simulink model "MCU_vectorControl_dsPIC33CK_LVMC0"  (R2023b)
settings: Solver=FixedStepDiscrete  StartTime=0.0  StopTime=10.0  FixedStep=5e-5  RelTol=1e-3  EnableMultiTasking=on
undefined symbols (not defined in the file or in its folder): A0, A4, ADC, address, also, AN0, AN1, as, B0, B2, below, Bias1, Bias2, bit, bits, BOR, C12, C13, C14, C7, C8, cause, Code, Communicate, control, counter, Custom, D11, D12, D13, D14, D2, D5, D6, D7, D9, dead, default, deviced, diff, disasserted, DiscIntNeverNeededParam, ECIO, ensure, events, faster, HS3, I, I2C, I2C1, I2C2, I2C3, illegalInstruction, Interval, inverter, is, IsSigned1, IsSigned2, kHz, Lowest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
libraries: simulink x55, MCHP_Blockset x25
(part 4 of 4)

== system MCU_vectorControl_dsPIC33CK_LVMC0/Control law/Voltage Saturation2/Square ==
  In1 : Inport
  Data Type Propagation : simulink/Signal Attributes/Data Type Propagation  PropDataType=fixdt(1, 16)  IfRefDouble=double  IfRefSingle=single  IsSigned=IsSigned1 or IsSigned2  NumBitsBase=max([NumBits1 NumBits2])  NumBitsMult=1  NumBitsAdd=0  NumBitsAllowFinal=1:128  PropScalingMode=Specify via dialog  PropScaling=2^-model.FracLen.volt2  ValuesUsedBestPrec=[5 -7]  SlopeBase=PosRange1*PosRange2  SlopeMult=1  SlopeAdd=0  BiasBase=max([Bias1 Bias2])  BiasMult=1  BiasAdd=0
  Square : Math  Operator=square  OutDataTypeStr=Inherit: Inherit via back propagation
  y : Outport
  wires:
  Square/1 -> Data Type Propagation/3, y/1
  In1/1 -> Square/1, Data Type Propagation/2, Data Type Propagation/1

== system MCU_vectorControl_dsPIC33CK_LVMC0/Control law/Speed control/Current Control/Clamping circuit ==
  note: The clamping enable or disable the integral action.
  preIntegrator : Inport  DisableCoverage=on
  saturation : Inport  DisableCoverage=on  Port=2
  AND : Logic  Operator=OR  IconShape=distinctive  AllPortsSameDT=off  OutDataTypeStr=boolean
  Compare To Zero1 : simulink/Logic and Bit Operations/Compare To Zero  relop=<=  OutDataTypeStr=boolean
  Delay : Delay  DelayLength=1
  Demux : Demux  Outputs=2
  Multiply : Product
  Clamp : Outport  DisableCoverage=on  VectorParamsAs1DForOutWhenUnconnected=off
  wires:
  saturation/1 -> Delay/1
  Compare To Zero1/1 -> Demux/1
  Multiply/1 -> Compare To Zero1/1
  preIntegrator/1 -> Multiply/2
  AND/1 -> Clamp/1
  Demux/2 -> AND/2
  Demux/1 -> AND/1
  Delay/1 -> Multiply/1

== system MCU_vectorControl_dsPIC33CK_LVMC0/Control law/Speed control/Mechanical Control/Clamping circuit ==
  note: The clamping enable or disable the integral action.
  Saturation : Inport  DisableCoverage=on
  preIntegrator : Inport  DisableCoverage=on  Port=2
  Compare To Zero1 : simulink/Logic and Bit Operations/Compare To Zero  relop=<=  OutDataTypeStr=boolean
  Delay : Delay  DelayLength=1  InitialCondition=0
  Multiply : Product
  Clamp : Outport  DisableCoverage=on  VectorParamsAs1DForOutWhenUnconnected=off
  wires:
  Delay/1 -> Multiply/1
  Saturation/1 -> Delay/1
  Multiply/1 -> Compare To Zero1/1
  preIntegrator/1 -> Multiply/2
  Compare To Zero1/1 -> Clamp/1

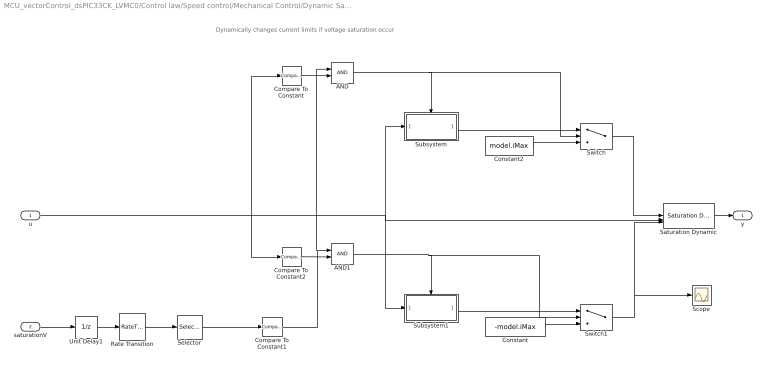
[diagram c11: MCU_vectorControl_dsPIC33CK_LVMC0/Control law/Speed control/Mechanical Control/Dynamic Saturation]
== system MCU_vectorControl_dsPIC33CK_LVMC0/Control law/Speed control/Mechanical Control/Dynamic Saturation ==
  note: Dynamically changes current limits if voltage saturation occur
  u : Inport
  saturationV : Inport  Port=2
  AND : Logic  IconShape=distinctive  AllPortsSameDT=off  OutDataTypeStr=boolean
  AND1 : Logic  IconShape=distinctive  AllPortsSameDT=off  OutDataTypeStr=boolean
  Compare To Constant : simulink/Logic and Bit Operations/Compare To Constant  relop=>=  const=0  OutDataTypeStr=boolean
  Compare To Constant1 : simulink/Logic and Bit Operations/Compare To Constant  relop=~=  const=0  OutDataTypeStr=boolean
  Compare To Constant2 : simulink/Logic and Bit Operations/Compare To Constant  relop=<  const=0  OutDataTypeStr=boolean
  Constant : Constant  Value=-model.iMax  OutDataTypeStr=single  SampleTime=1e-3
  Constant2 : Constant  Value=model.iMax  OutDataTypeStr=single  SampleTime=1e-3
  Rate Transition : RateTransition  OutPortSampleTime=control.tsMeca
  Saturation Dynamic : simulink/Discontinuities/Saturation Dynamic  OutMin=[]  OutMax=[]  OutDataTypeStr=Inherit: Same as second input  OutDataType=fixdt(1, 16)  OutScaling=2^-10  DoSatur=off
  Scope : Scope
  Selector : Selector  InputPortWidth=2  IndexOptions=Index vector (dialog)  Indices=2  OutputSizes=1
  Subsystem : Subsystem
  Subsystem1 : Subsystem
  Switch : Switch  Criteria=u2 > Threshold
  Switch1 : Switch  Criteria=u2 > Threshold
  Unit Delay1 : UnitDelay  SampleTime=-1  HasFrameUpgradeWarning=on
  y : Outport
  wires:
  Switch/1 -> Saturation Dynamic/1
  u/1 -> Compare To Constant/1, Compare To Constant2/1, Subsystem/1(u), Subsystem1/1(u), Saturation Dynamic/2
  Saturation Dynamic/1 -> y/1
  saturationV/1 -> Unit Delay1/1
  Compare To Constant1/1 -> AND/1, AND1/1
  AND/1 -> Switch/2, Subsystem/Trigger
  Constant2/1 -> Switch/3
  Subsystem/1(Out1) -> Switch/1
  Compare To Constant2/1 -> AND1/2
  AND1/1 -> Subsystem1/Trigger, Switch1/2
  Subsystem1/1(Out1) -> Switch1/1
  Switch1/1 -> Scope/1, Saturation Dynamic/3
  Constant/1 -> Switch1/3
  Rate Transition/1 -> Selector/1
  Unit Delay1/1 -> Rate Transition/1
  Compare To Constant/1 -> AND/2
  Selector/1 -> Compare To Constant1/1

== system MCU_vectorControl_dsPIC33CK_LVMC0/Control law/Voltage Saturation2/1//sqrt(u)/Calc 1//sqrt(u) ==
  u : Inport
  Enable : EnablePort
  Reciprocal : Product  Inputs=/
  Sqrt : Sqrt
  Out1 : Outport
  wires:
  Reciprocal/1 -> Out1/1
  u/1 -> Sqrt/1
  Sqrt/1 -> Reciprocal/1

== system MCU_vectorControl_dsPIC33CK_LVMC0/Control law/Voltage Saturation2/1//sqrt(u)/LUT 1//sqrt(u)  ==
  y : Inport
  Enable : EnablePort
  1-D Lookup Table : Lookup_n-D  NumberOfTableDimensions=1  BreakpointsSpecification=Even spacing  BreakpointsForDimension1=model.math.LUTintsqrtx  BreakpointsForDimension1FirstPoint=model.math.LUTintsqrtx(1)  BreakpointsForDimension1Spacing=mean(diff(model.math.LUTintsqrtx))  IndexSearchMethod=Evenly spaced points  Table=model.math.LUTintsqrty  ExtrapMethod=Clip  DiagnosticForOutOfRangeInput=Error  UseLastTableValue=on  InternalRulePriority=Speed  OutDataTypeStr=Inherit: Inherit via back propagation  RndMeth=Simplest  FractionDataTypeStr=fixdt(1,16,15)
  Data Type Propagation : simulink/Signal Attributes/Data Type Propagation  PropDataType=fixdt(1, 16)  IfRefDouble=double  IfRefSingle=single  IsSigned=IsSigned1 or IsSigned2  NumBitsBase=max([NumBits1 NumBits2])  NumBitsMult=1  NumBitsAdd=0  NumBitsAllowFinal=1:128  PropScalingMode=Specify via dialog  PropScaling=2^-model.FracLen.invsqrtvolt  ValuesUsedBestPrec=[5 -7]  SlopeBase=PosRange1*PosRange2  SlopeMult=1  SlopeAdd=0  BiasBase=max([Bias1 Bias2])  BiasMult=1  BiasAdd=0
  vdqsat1 : Outport
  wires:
  1-D Lookup Table/1 -> Data Type Propagation/3, vdqsat1/1
  y/1 -> 1-D Lookup Table/1, Data Type Propagation/2, Data Type Propagation/1

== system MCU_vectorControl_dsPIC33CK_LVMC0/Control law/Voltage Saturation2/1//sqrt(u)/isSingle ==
  u : Inport
  Compare To Constant : simulink/Logic and Bit Operations/Compare To Constant  relop=>=  const=500000  OutDataTypeStr=boolean
  Constant1 : Constant  OutDataTypeStr=Inherit: Inherit via back propagation
  Data Type Duplicate : DataTypeDuplicate
  Data Type Propagation : simulink/Signal Attributes/Data Type Propagation  PropDataType=fixdt(1, 16)  IfRefDouble=double  IfRefSingle=single  IsSigned=IsSigned1 or IsSigned2  NumBitsBase=max([NumBits1 NumBits2])  NumBitsMult=1  NumBitsAdd=0  NumBitsAllowFinal=1:128  PropScaling=2^-10  ValuesUsedBestPrec=[5 -7]  SlopeBase=max([PosRange1 PosRange2])  SlopeMult=100000  SlopeAdd=0  BiasBase=Bias1  BiasMult=1  BiasAdd=0
  Data Type Conversion : DataTypeConversion
  Gain : Gain  Gain=10000  SaturateOnIntegerOverflow=on
  y : Outport
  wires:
  u/1 -> Data Type Duplicate/1
  Constant1/1 -> Gain/1, Data Type Duplicate/2
  Gain/1 -> Data Type Conversion/1, Data Type Propagation/2, Data Type Propagation/1
  Data Type Conversion/1 -> Data Type Propagation/3, Compare To Constant/1
  Compare To Constant/1 -> y/1

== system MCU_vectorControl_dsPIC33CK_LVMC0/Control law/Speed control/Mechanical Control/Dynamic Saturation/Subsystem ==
  u : Inport
  Trigger : TriggerPort  VariantControl=(inherit)  PortDimensions=1
  Out1 : Outport
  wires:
  u/1 -> Out1/1

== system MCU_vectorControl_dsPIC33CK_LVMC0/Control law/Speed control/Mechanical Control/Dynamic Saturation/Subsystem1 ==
  u : Inport
  Trigger : TriggerPort  VariantControl=(inherit)  PortDimensions=1
  Out1 : Outport
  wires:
  u/1 -> Out1/1
